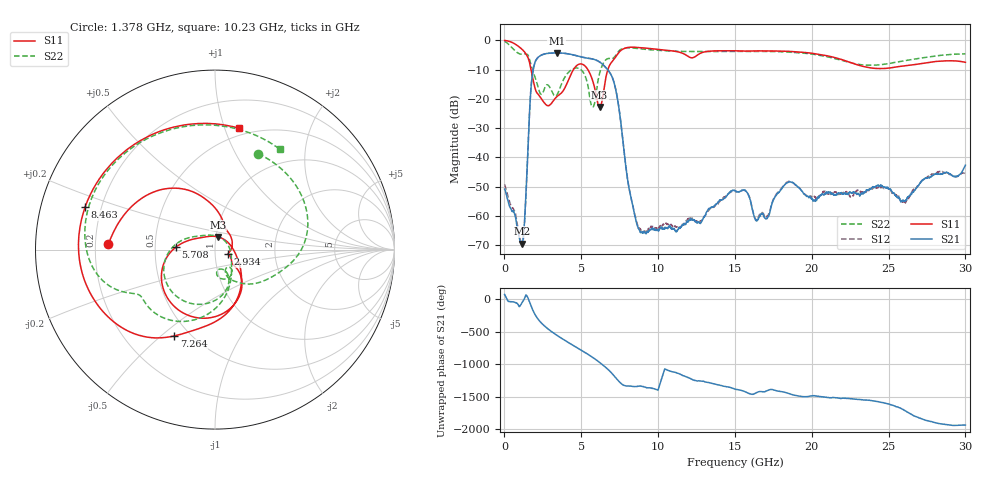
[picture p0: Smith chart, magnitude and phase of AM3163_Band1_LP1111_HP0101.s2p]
!Agilent Technologies,E8364B,MY43040894,A.07.50.67
!Agilent E8364B: A.07.50.67
!Date: Thursday, August 20, 2020 11:58:24
!Correction: S11(Full 2 Port(1,2))
!S21(Full 2 Port(1,2))
!S12(Full 2 Port(1,2))
!S22(Full 2 Port(1,2))
!S2P File: Measurements: S11, S21, S12, S22:
# Hz S  dB  R 50
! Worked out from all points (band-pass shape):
!   3201 points, 10 MHz to 30 GHz, reference 50 ohm
!   highest |S21| = -4.30 dB at 3.403 GHz (marker M1); lowest = -69.4 dB at 1.135 GHz (marker M2)
!   |S21| within 3 dB of the highest: 2.004 GHz to 6.168 GHz (4.163 GHz wide, 102 % of centre)
!   lowest |S11| = -22.8 dB at 6.186 GHz (marker M3), VSWR 1.16, Z = 51.1 + j7.29 ohm
!   |S11| at or under -10 dB: 1.726 GHz to 4.491 GHz (2.765 GHz wide, 88.9 % of centre); 5.428 GHz to 6.73 GHz (1.302 GHz wide, 21.4 % of centre)
!   |S22| runs from -22.8 to -0.4 dB; largest |S21 - S12| = 0.004
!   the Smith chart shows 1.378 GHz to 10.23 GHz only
!   S11 on the Smith chart (normalised r, x): 1.378 GHz: 0.25, +0.02; 2.934 GHz: 1.16, -0.06; 5.708 GHz: 0.64, +0.02; 7.264 GHz: 0.41, -0.55; 8.463 GHz: 0.14, +0.16; 10.23 GHz: 0.44, +1.12
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1e7  -0.05 -8.1  -50.82 76.1  -49.17 -1.7  -0.37 -15.0
4.5985e8  -0.64 -56.2  -58.03 -33.7  -56.74 -28.9  -2.36 -96.1
1.134625e9  -3.03 -143.6  -69.37 -52.7  -69.93 28.7  -4.74 124.2
1.378294e9  -4.51 177.1  -54.62 61.3  -55.46 88.5  -4.65 65.8
1.875003e9  -13.77 84.0  -9.92 -178.8  -9.93 -179.0  -10.73 -40.6
2.418572e9  -20.04 15.5  -5.01 -5.9  -5.02 -5.9  -18.43 -55.6
2.934025e9  -22.16 -19.1  -4.39 -111.8  -4.41 -111.8  -15.88 -80.4
3.402619e9  -19.27 -32.5  -4.30 170.2  -4.32 170.2  -18.73 -70.1
4.011791e9  -15.37 -41.5  -4.50 78.2  -4.53 78.3  -11.92 -80.1
5.014581e9  -8.08 -119.0  -5.70 -64.4  -5.68 -64.1  -10.20 -157.4
5.7081e9  -13.26 176.1  -6.37 -166.9  -6.34 -167.0  -22.70 68.8
6.186066e9  -22.76 77.4  -7.36 111.1  -7.40 111.0  -11.38 -78.5
7.263831e9  -5.49 -115.2  -17.34 -132.4  -17.32 -131.8  -5.02 -155.1
8.463431e9  -2.37 161.8  -59.40 98.2  -58.98 101.0  -2.69 131.9
1.000979e10  -3.11 88.3  -64.87 53.3  -64.21 37.7  -3.44 65.6
1.023472e10  -3.23 78.7  -64.39 -136.6  -63.43 20.1  -3.53 56.9
1.5005e10  -3.59 -71.9  -51.32 58.8  -51.51 61.8  -3.79 -92.5
1.641078e10  -3.62 -105.8  -61.58 3.4  -61.32 8.4  -3.79 -126.9
2.000958e10  -4.42 162.8  -53.99 -46.1  -53.56 -49.3  -4.71 135.4
2.274617e10  -7.98 59.8  -51.77 -93.9  -52.12 -96.4  -7.92 20.3
2.500479e10  -9.49 -63.0  -50.74 -170.3  -50.64 -170.7  -7.97 -93.2
3e10  -7.50 104.9  -42.65 -134.8  -45.52 -130.2  -4.61 100.4
